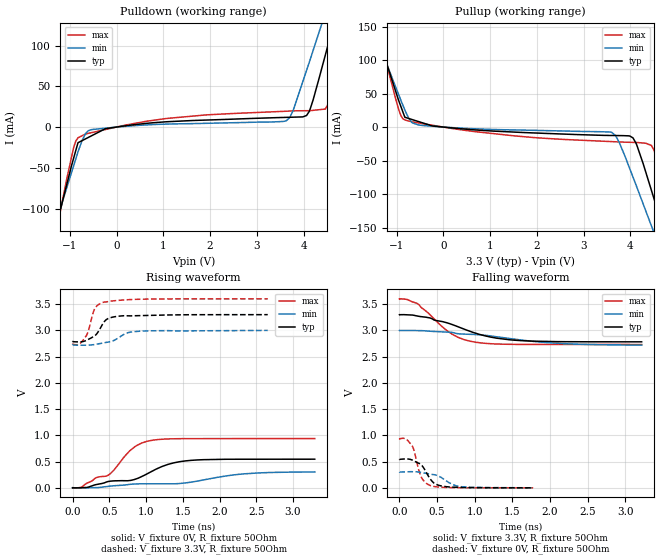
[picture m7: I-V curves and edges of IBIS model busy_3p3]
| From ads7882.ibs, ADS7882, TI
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|   busy_3p3 Model
[Model]   busy_3p3
Model_type   Output
Polarity   Non-Inverting
Vmeas = 1.65
Vref = 1.65
Cref = 20pF
Rref = 50
|   typ   min   max
|   (nom PVT)   (Fast PVT)   (slow PVT)
|C_comp from frequency sweep method (F=1.5MHz)
C_comp   1.164e-12   1.043e-12   1.312e-12
|ON state : BUFFER OUTPUT TURNED HIGH
|C_comp   1.164e-12   1.043e-12   1.312e-12
|OFF state: BUFFER OUTPUT TURNED LOW
|C_comp   1.201e-12   1.064e-12   1.341e-12
|C_comp from LC tank measurement(L=1nH)
|Resonant Frequency(Hz)   5.950e+09   6.040e+09   5.790e+09
|C_comp   7.162e-13   6.950e-13   7.564e-13
|ON state : BUFFER OUTPUT TURNED HIGH
|Resonant Frequency(Hz)   5.950e+09   6.040e+09   5.790e+09
|C_comp   7.162e-13   6.950e-13   7.564e-13
|OFF state: BUFFER IN HIGH IMPEDANCE
|Resonant Frequency   5.970e+09   6.030e+09   5.340e+09
|C_comp   7.114e-13   6.973e-13   8.892e-13
| Where nom  PVT is Nominal Process,  3.3V,  25C
|   Fast PVT is Strong Process,   3.6V,  -40C
|   Slow PVT is Weak Process,   3V,  85C
[Voltage Range]   3.3   3   3.6
|Ambient Temperature   25   85   -40
|Junction Temperature
[Temperature Range]   25   85   -40
[Pullup Reference]   3.3   3   3.6
[Pulldown Reference]   0   0   0
[Power Clamp Reference]   3.3   3   3.6
[GND Clamp Reference]   0   0   0
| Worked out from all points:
|   slope of the pulldown table from 0 to 0.495 V, typ, clamps not added: 135 ohm
|   slope of the pullup table from 0 to 0.495 V, typ, clamps not added: 154 ohm
|   falling waveform, V_fixture 3.3V, R_fixture 50Ohm: 20-80 % time 704ps typ, 1.13ns min, 431ps max; typ from 3.3 V to 2.78 V
|   rising waveform, V_fixture 0V, R_fixture 50Ohm: 20-80 % time 821ps typ, 1.42ns min, 505ps max; typ from 0 V to 0.545 V
|   rising waveform, V_fixture 3.3V, R_fixture 50Ohm: 20-80 % time 161ps typ, 254ps min, 118ps max; typ from 2.78 V to 3.3 V
|   falling waveform, V_fixture 0V, R_fixture 50Ohm: 20-80 % time 154ps typ, 224ps min, 112ps max; typ from 0.546 V to 0.001 V
[Pulldown]
|   Voltage   I(typ)   I(min)   I(max)
-3.3V     -584.2mA   -489.9mA   -713.8mA
-1.313V   -126.9mA   -120.2mA   -135.5mA
-870mV    -28.39mA   -38.76mA   -16.97mA
-537mV    -10.76mA   -3.157mA   -6.865mA
640.2mV   4.559mA    2.647mA    7.129mA
3.633V    11.91mA    7.782mA    19.45mA
4.122V    19.14mA    79.21mA    20.09mA
4.336V    60.44mA    117.1mA    21.32mA
4.465V    87.99mA    139.9mA    22.11mA
4.584V    113.4mA    160.9mA    40.74mA
5.2V      244.9mA    269.6mA    201.3mA
6.6V      544mA      517mA      570.5mA
[Pullup]
|   Voltage   I(typ)   I(min)   I(max)
-3.3V     545.2mA    465.2mA    650.7mA
-1.01V    51.01mA    57.88mA    39.33mA
-823.2mV  14.6mA     25.08mA    10.52mA
-669mV    11.21mA    6.467mA    7.819mA
-438mV    6.121mA    2.303mA    5.051mA
3.594V    -12.56mA   -7.762mA   -21.7mA
3.986V    -13.33mA   -62.03mA   -22.73mA
4.138V    -27.06mA   -89.68mA   -22.99mA
4.451V    -94.59mA   -147.6mA   -27.58mA
4.696V    -149.8mA   -193.1mA   -83.39mA
5.25V     -276.5mA   -295.8mA   -240.8mA
6.6V      -585.2mA   -546.2mA   -630.9mA
[Ramp]
R_load = 50
|   typ   min   max
dV/dt_r   0.327706/8.21559e-10   0.182124/1.41923e-09   0.563074/5.04922e-10
dV/dt_f   0.310196/7.04693e-10   0.168528/1.14639e-09   0.520808/4.31951e-10
[Falling Waveform]
V_fixture = 3.3V
V_fixture_min = 3V
V_fixture_max = 3.6V
R_fixture = 50Ohm
|   Time   V(typ)   V(min)   V(max)
0s        3.3V       3V         3.6V
101.4ps   3.298V     3.001V     3.59V
249.2ps   3.272V     2.997V     3.503V
629.5ps   3.147V     2.969V     2.998V
776ps     3.072V     2.939V     2.871V
936ps     2.984V     2.927V     2.796V
1.216ns   2.872V     2.894V     2.748V
1.616ns   2.806V     2.818V     2.734V
2.256ns   2.786V     2.744V     2.734V
3.216ns   2.783V     2.721V     2.733V
[Rising Waveform]
V_fixture = 0V
V_fixture_min = 0V
V_fixture_max = 0V
R_fixture = 50Ohm
|   Time   V(typ)   V(min)   V(max)
0s        1.565nV    6.201nV    1.48nV
119.2ps   1.329mV    -140.3uV   11.04mV
317.5ps   60.29mV    3.418mV    190.2mV
484.1ps   119.7mV    27mV       238.9mV
776ps     138.5mV    64.82mV    702mV
1.016ns   267.3mV    75.87mV    886.8mV
1.296ns   445mV      75.86mV    930.8mV
1.616ns   523.3mV    108.2mV    936.8mV
2.336ns   544.2mV    265.8mV    937.3mV
3.296ns   545.4mV    302mV      938mV
[Rising Waveform]
V_fixture = 3.3V
V_fixture_min = 3V
V_fixture_max = 3.6V
R_fixture = 50Ohm
|   Time   V(typ)   V(min)   V(max)
0s        2.783V     2.719V     2.732V
101.4ps   2.78V      2.717V     2.749V
182.3ps   2.806V     2.716V     2.887V
215.1ps   2.828V     2.719V     2.993V
299.8ps   2.893V     2.73V      3.408V
431.8ps   3.166V     2.763V     3.54V
570.8ps   3.259V     2.813V     3.564V
752.2ps   3.277V     2.955V     3.584V
871ps     3.279V     2.979V     3.591V
2.656ns   3.299V     2.999V     3.6V
[Falling Waveform]
V_fixture = 0V
V_fixture_min = 0V
V_fixture_max = 0V
R_fixture = 50Ohm
|   Time   V(typ)   V(min)   V(max)
0s        546.1mV    303.8mV    938.4mV
86.69ps   552.5mV    306.4mV    931.7mV
163.7ps   533.8mV    308.7mV    815.3mV
190.6ps   516.4mV    307.9mV    726.7mV
283.3ps   446.9mV    296.7mV    226.2mV
334.7ps   350.7mV    282.3mV    114.6mV
407.8ps   171.3mV    262.6mV    46.38mV
508.1ps   55.61mV    232.7mV    17.77mV
795.9ps   9.881mV    27.3mV     3.131mV
1.776ns   1.46mV     2.014mV    1.046mV
